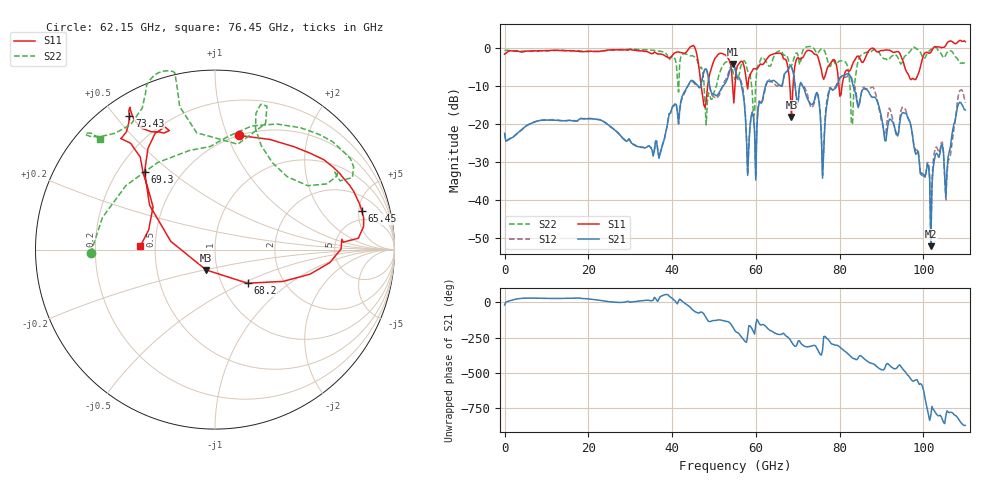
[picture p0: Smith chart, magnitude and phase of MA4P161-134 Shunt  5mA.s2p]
!Keysight Technologies,N5247B,US61255204,A.15.70.20
!Date: Friday, October 21, 2022 14:13:07
!Correction: S11(C  4-Port  )
!S31(C  4-Port  )
!S13(C  4-Port  )
!S33(C  4-Port  )
!S2P File: Measurements: S11, S31, S13, S33:
# Hz S  dB  R 50
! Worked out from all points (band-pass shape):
!   401 points, 10 MHz to 110 GHz, reference 50 ohm
!   highest |S21| = -4.29 dB at 54.46 GHz (marker M1); lowest = -52.0 dB at 101.8 GHz (marker M2)
!   |S21| within 3 dB of the highest: 53.46 GHz to 55.44 GHz (1.983 GHz wide, 3.64 % of centre); 66.75 GHz to 69.03 GHz (2.283 GHz wide, 3.36 % of centre)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
!   lowest |S11| = -18.1 dB at 68.48 GHz (marker M3), VSWR 1.28, Z = 44.2 - j10.2 ohm
!   |S11| at or under -10 dB: 46.93 GHz to 48.49 GHz (1.567 GHz wide, 3.28 % of centre); 54.45 GHz to 55 GHz (554.5 MHz wide, 1.01 % of centre); 68.09 GHz to 68.87 GHz (774.6 MHz wide, 1.13 % of centre)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
!   |S22| runs from -20.2 to 0.3 dB; largest |S21 - S12| = 0.16
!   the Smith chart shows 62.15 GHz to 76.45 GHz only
!   S11 on the Smith chart (normalised r, x): 62.15 GHz: 0.50, +1.11; 65.45 GHz: 3.61, +5.43; 68.2 GHz: 1.32, -0.53; 69.3 GHz: 0.31, +0.41; 73.43 GHz: 0.08, +0.55; 76.45 GHz: 0.41, +0.02
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1e7  -1.72 -178.5  -22.44 -17.7  -22.41 -17.5  -0.79 -178.6
1.843332e10  -1.04 130.7  -18.58 28.6  -18.59 28.5  -0.89 140.5
3.685665e10  -1.64 126.3  -28.96 26.8  -28.83 27.0  -0.89 133.7
4.565585e10  -0.70 52.2  -9.38 -68.5  -9.77 -66.9  -2.75 27.0
5.445505e10  -10.10 98.2  -4.29 -174.2  -4.35 -173.9  -5.96 127.5
5.5005e10  -9.97 -177.5  -5.33 158.6  -5.55 158.2  -8.29 148.0
5.802972e10  -10.83 159.3  -33.49 128.1  -33.30 128.2  -6.13 167.5
6.077948e10  -4.70 149.6  -14.31 -149.7  -13.95 -150.6  -4.15 -121.8
6.215435e10  -3.74 77.9  -10.52 -165.0  -11.21 -159.4  -3.18 -178.3
6.545405e10  -1.46 14.7  -9.68 132.0  -9.70 153.9  -0.93 37.9
6.82038e10  -11.67 -45.9  -4.77 93.0  -4.94 90.1  -4.86 45.2
6.847878e10  -18.15 -113.4  -4.96 79.7  -5.15 77.4  -4.73 56.5
6.93037e10  -4.66 132.1  -9.54 47.9  -9.28 47.3  -2.02 73.3
7.342832e10  -1.06 122.6  -14.89 51.3  -15.73 49.5  0.11 111.0
7.645305e10  -7.59 177.6  -20.36 118.5  -19.38 130.6  -1.01 136.0
8.085265e10  -8.18 -75.9  -7.24 20.6  -7.67 21.1  -3.50 -144.1
8.305245e10  -4.35 -45.6  -9.33 -36.9  -8.78 -20.7  -20.11 11.4
8.607718e10  -2.77 6.3  -10.87 -47.4  -10.72 -46.1  -1.28 -14.9
9.185165e10  -0.67 71.6  -18.77 -86.1  -15.83 -83.0  -3.01 67.1
9.762612e10  -8.17 177.7  -25.30 158.7  -24.90 156.8  0.14 165.9
1.017508e11  -1.19 -88.1  -52.03 -86.6  -51.83 -91.0  -0.50 -124.6
1.1e11  1.53 8.1  -16.33 -156.9  -14.42 -161.4  -4.06 16.6
